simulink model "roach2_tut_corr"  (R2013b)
settings: Solver=VariableStepDiscrete  SolverMode=SingleTasking  StartTime=0.0  StopTime=100  RelTol=1e-3
undefined symbols (not defined in the file): add_latency, addr_width, Bit, bitfield, BitWidth, bram_latency, burst_size, casper_library_scopes, conv_latency, data_width, DelayLen, fan_latency, FFTSize, FFTStage, getfield, increment, led, Location, Lower, mult_latency, mux_latency, n_bits, n_bits_data, n_inputs, n_streams, n_taps, neg_latency, negate_latency, nsamples, pfb_size, pulse_len, reset_period, ROACH, ROACH2, snapshot, sx475t, sync_period, sync_period_bits, Upper, UseCounter, Width
libraries: xbsIndex_r4 x24444, casper_library_misc x73, xbsReplacements_r4 x34, casper_library_delays x14, xps_library x7
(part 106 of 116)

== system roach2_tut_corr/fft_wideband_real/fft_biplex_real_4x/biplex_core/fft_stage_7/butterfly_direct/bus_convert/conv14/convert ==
  note: (ones_bit & 1) -> round-to-even (ones_bit ^ 1) -> round-to-odd (sign_bit & 1)-> round-to-zero (sign_bit ^ 1) -> round-to-inf (X ~| 1) -> round half down (X | 1) -> round half up
  in : Inport
  Concat : xbsIndex_r4/Concat  num_inputs=2  dbl_ovrd=off  block_type=concat
  Constant : xbsIndex_r4/Constant  const=1  gui_display_data_type=Fixed-point  arith_type=Unsigned  n_bits=1  bin_pt=0  preci_type=Single  exp_width=8  frac_width=24  explicit_period=off  period=1  equ=P=C  opselect=C  inp2=PCIN>>17  opr=+  inp1=P  carry=CIN  dbl_ovrd=off  block_type=constant
  Reinterpret : xbsIndex_r4/Reinterpret  force_arith_type=on  arith_type=Unsigned  force_bin_pt=on  bin_pt=0  block_type=reinterpret
  adder : xbsIndex_r4/AddSub  mode=Addition  use_carryin=off  use_carryout=off  en=off  latency=1  precision=User Defined  arith_type="Signed  (2's comp)"  n_bits=18  bin_pt=17  quantization=Truncate  overflow=Wrap  dbl_ovrd=off  use_behavioral_HDL=off  hw_selection=Fabric  pipelined=on  use_rpm=on  block_type=addsub
  almost_half : xbsIndex_r4/Constant  const=1  gui_display_data_type=Fixed-point  arith_type=Unsigned  n_bits=19  bin_pt=0  preci_type=Single  exp_width=8  frac_width=24  explicit_period=off  period=1  equ=P=C  opselect=C  inp2=PCIN>>17  opr=+  inp1=P  carry=CIN  dbl_ovrd=off  block_type=constant
  bit : xbsIndex_r4/Slice  nbits=1  boolean_output=off  mode=Lower Bit Location + Width  bit1=0  base1=MSB of Input  bit0=1  base0=LSB of Input  dbl_ovrd=off  block_type=slice
  force1 : xbsIndex_r4/Reinterpret  force_arith_type=on  arith_type="Signed  (2's comp)"  force_bin_pt=on  bin_pt=19  block_type=reinterpret
  force2 : xbsIndex_r4/Reinterpret  force_arith_type=off  arith_type="Signed  (2's comp)"  force_bin_pt=on  bin_pt=19  block_type=reinterpret
  tweak_op : xbsIndex_r4/Logical  logical_function=AND  inputs=2  en=off  latency=0  precision=Full  arith_type=Unsigned  n_bits=8  bin_pt=2  align_bp=on  dbl_ovrd=off  block_type=logical
  out : Outport
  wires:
  tweak_op/1 -> Concat/2
  Constant/1 -> tweak_op/2
  bit/1 -> tweak_op/1
  almost_half/1 -> force2/1
  in/1 -> Reinterpret/1, bit/1
  Concat/1 -> force1/1
  Reinterpret/1 -> Concat/1
  force1/1 -> adder/1
  force2/1 -> adder/2
  adder/1 -> out/1

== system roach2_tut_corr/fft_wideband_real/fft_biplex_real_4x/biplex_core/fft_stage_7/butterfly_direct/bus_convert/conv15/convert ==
  note: (ones_bit & 1) -> round-to-even (ones_bit ^ 1) -> round-to-odd (sign_bit & 1)-> round-to-zero (sign_bit ^ 1) -> round-to-inf (X ~| 1) -> round half down (X | 1) -> round half up
  in : Inport
  Concat : xbsIndex_r4/Concat  num_inputs=2  dbl_ovrd=off  block_type=concat
  Constant : xbsIndex_r4/Constant  const=1  gui_display_data_type=Fixed-point  arith_type=Unsigned  n_bits=1  bin_pt=0  preci_type=Single  exp_width=8  frac_width=24  explicit_period=off  period=1  equ=P=C  opselect=C  inp2=PCIN>>17  opr=+  inp1=P  carry=CIN  dbl_ovrd=off  block_type=constant
  Reinterpret : xbsIndex_r4/Reinterpret  force_arith_type=on  arith_type=Unsigned  force_bin_pt=on  bin_pt=0  block_type=reinterpret
  adder : xbsIndex_r4/AddSub  mode=Addition  use_carryin=off  use_carryout=off  en=off  latency=1  precision=User Defined  arith_type="Signed  (2's comp)"  n_bits=18  bin_pt=17  quantization=Truncate  overflow=Wrap  dbl_ovrd=off  use_behavioral_HDL=off  hw_selection=Fabric  pipelined=on  use_rpm=on  block_type=addsub
  almost_half : xbsIndex_r4/Constant  const=1  gui_display_data_type=Fixed-point  arith_type=Unsigned  n_bits=19  bin_pt=0  preci_type=Single  exp_width=8  frac_width=24  explicit_period=off  period=1  equ=P=C  opselect=C  inp2=PCIN>>17  opr=+  inp1=P  carry=CIN  dbl_ovrd=off  block_type=constant
  bit : xbsIndex_r4/Slice  nbits=1  boolean_output=off  mode=Lower Bit Location + Width  bit1=0  base1=MSB of Input  bit0=1  base0=LSB of Input  dbl_ovrd=off  block_type=slice
  force1 : xbsIndex_r4/Reinterpret  force_arith_type=on  arith_type="Signed  (2's comp)"  force_bin_pt=on  bin_pt=19  block_type=reinterpret
  force2 : xbsIndex_r4/Reinterpret  force_arith_type=off  arith_type="Signed  (2's comp)"  force_bin_pt=on  bin_pt=19  block_type=reinterpret
  tweak_op : xbsIndex_r4/Logical  logical_function=AND  inputs=2  en=off  latency=0  precision=Full  arith_type=Unsigned  n_bits=8  bin_pt=2  align_bp=on  dbl_ovrd=off  block_type=logical
  out : Outport
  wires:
  tweak_op/1 -> Concat/2
  Constant/1 -> tweak_op/2
  bit/1 -> tweak_op/1
  almost_half/1 -> force2/1
  in/1 -> Reinterpret/1, bit/1
  Concat/1 -> force1/1
  Reinterpret/1 -> Concat/1
  force1/1 -> adder/1
  force2/1 -> adder/2
  adder/1 -> out/1

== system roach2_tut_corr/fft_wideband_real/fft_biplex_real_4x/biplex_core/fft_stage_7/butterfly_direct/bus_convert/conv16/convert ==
  note: (ones_bit & 1) -> round-to-even (ones_bit ^ 1) -> round-to-odd (sign_bit & 1)-> round-to-zero (sign_bit ^ 1) -> round-to-inf (X ~| 1) -> round half down (X | 1) -> round half up
  in : Inport
  Concat : xbsIndex_r4/Concat  num_inputs=2  dbl_ovrd=off  block_type=concat
  Constant : xbsIndex_r4/Constant  const=1  gui_display_data_type=Fixed-point  arith_type=Unsigned  n_bits=1  bin_pt=0  preci_type=Single  exp_width=8  frac_width=24  explicit_period=off  period=1  equ=P=C  opselect=C  inp2=PCIN>>17  opr=+  inp1=P  carry=CIN  dbl_ovrd=off  block_type=constant
  Reinterpret : xbsIndex_r4/Reinterpret  force_arith_type=on  arith_type=Unsigned  force_bin_pt=on  bin_pt=0  block_type=reinterpret
  adder : xbsIndex_r4/AddSub  mode=Addition  use_carryin=off  use_carryout=off  en=off  latency=1  precision=User Defined  arith_type="Signed  (2's comp)"  n_bits=18  bin_pt=17  quantization=Truncate  overflow=Wrap  dbl_ovrd=off  use_behavioral_HDL=off  hw_selection=Fabric  pipelined=on  use_rpm=on  block_type=addsub
  almost_half : xbsIndex_r4/Constant  const=1  gui_display_data_type=Fixed-point  arith_type=Unsigned  n_bits=19  bin_pt=0  preci_type=Single  exp_width=8  frac_width=24  explicit_period=off  period=1  equ=P=C  opselect=C  inp2=PCIN>>17  opr=+  inp1=P  carry=CIN  dbl_ovrd=off  block_type=constant
  bit : xbsIndex_r4/Slice  nbits=1  boolean_output=off  mode=Lower Bit Location + Width  bit1=0  base1=MSB of Input  bit0=1  base0=LSB of Input  dbl_ovrd=off  block_type=slice
  force1 : xbsIndex_r4/Reinterpret  force_arith_type=on  arith_type="Signed  (2's comp)"  force_bin_pt=on  bin_pt=19  block_type=reinterpret
  force2 : xbsIndex_r4/Reinterpret  force_arith_type=off  arith_type="Signed  (2's comp)"  force_bin_pt=on  bin_pt=19  block_type=reinterpret
  tweak_op : xbsIndex_r4/Logical  logical_function=AND  inputs=2  en=off  latency=0  precision=Full  arith_type=Unsigned  n_bits=8  bin_pt=2  align_bp=on  dbl_ovrd=off  block_type=logical
  out : Outport
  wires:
  tweak_op/1 -> Concat/2
  Constant/1 -> tweak_op/2
  bit/1 -> tweak_op/1
  almost_half/1 -> force2/1
  in/1 -> Reinterpret/1, bit/1
  Concat/1 -> force1/1
  Reinterpret/1 -> Concat/1
  force1/1 -> adder/1
  force2/1 -> adder/2
  adder/1 -> out/1

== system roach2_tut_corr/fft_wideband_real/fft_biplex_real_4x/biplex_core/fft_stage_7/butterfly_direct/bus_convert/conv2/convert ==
  note: (ones_bit & 1) -> round-to-even (ones_bit ^ 1) -> round-to-odd (sign_bit & 1)-> round-to-zero (sign_bit ^ 1) -> round-to-inf (X ~| 1) -> round half down (X | 1) -> round half up
  in : Inport
  Concat : xbsIndex_r4/Concat  num_inputs=2  dbl_ovrd=off  block_type=concat
  Constant : xbsIndex_r4/Constant  const=1  gui_display_data_type=Fixed-point  arith_type=Unsigned  n_bits=1  bin_pt=0  preci_type=Single  exp_width=8  frac_width=24  explicit_period=off  period=1  equ=P=C  opselect=C  inp2=PCIN>>17  opr=+  inp1=P  carry=CIN  dbl_ovrd=off  block_type=constant
  Reinterpret : xbsIndex_r4/Reinterpret  force_arith_type=on  arith_type=Unsigned  force_bin_pt=on  bin_pt=0  block_type=reinterpret
  adder : xbsIndex_r4/AddSub  mode=Addition  use_carryin=off  use_carryout=off  en=off  latency=1  precision=User Defined  arith_type="Signed  (2's comp)"  n_bits=18  bin_pt=17  quantization=Truncate  overflow=Wrap  dbl_ovrd=off  use_behavioral_HDL=off  hw_selection=Fabric  pipelined=on  use_rpm=on  block_type=addsub
  almost_half : xbsIndex_r4/Constant  const=1  gui_display_data_type=Fixed-point  arith_type=Unsigned  n_bits=19  bin_pt=0  preci_type=Single  exp_width=8  frac_width=24  explicit_period=off  period=1  equ=P=C  opselect=C  inp2=PCIN>>17  opr=+  inp1=P  carry=CIN  dbl_ovrd=off  block_type=constant
  bit : xbsIndex_r4/Slice  nbits=1  boolean_output=off  mode=Lower Bit Location + Width  bit1=0  base1=MSB of Input  bit0=1  base0=LSB of Input  dbl_ovrd=off  block_type=slice
  force1 : xbsIndex_r4/Reinterpret  force_arith_type=on  arith_type="Signed  (2's comp)"  force_bin_pt=on  bin_pt=19  block_type=reinterpret
  force2 : xbsIndex_r4/Reinterpret  force_arith_type=off  arith_type="Signed  (2's comp)"  force_bin_pt=on  bin_pt=19  block_type=reinterpret
  tweak_op : xbsIndex_r4/Logical  logical_function=AND  inputs=2  en=off  latency=0  precision=Full  arith_type=Unsigned  n_bits=8  bin_pt=2  align_bp=on  dbl_ovrd=off  block_type=logical
  out : Outport
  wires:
  tweak_op/1 -> Concat/2
  Constant/1 -> tweak_op/2
  bit/1 -> tweak_op/1
  almost_half/1 -> force2/1
  in/1 -> Reinterpret/1, bit/1
  Concat/1 -> force1/1
  Reinterpret/1 -> Concat/1
  force1/1 -> adder/1
  force2/1 -> adder/2
  adder/1 -> out/1

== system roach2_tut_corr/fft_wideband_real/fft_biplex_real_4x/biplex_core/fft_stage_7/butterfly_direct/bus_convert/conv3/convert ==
  note: (ones_bit & 1) -> round-to-even (ones_bit ^ 1) -> round-to-odd (sign_bit & 1)-> round-to-zero (sign_bit ^ 1) -> round-to-inf (X ~| 1) -> round half down (X | 1) -> round half up
  in : Inport
  Concat : xbsIndex_r4/Concat  num_inputs=2  dbl_ovrd=off  block_type=concat
  Constant : xbsIndex_r4/Constant  const=1  gui_display_data_type=Fixed-point  arith_type=Unsigned  n_bits=1  bin_pt=0  preci_type=Single  exp_width=8  frac_width=24  explicit_period=off  period=1  equ=P=C  opselect=C  inp2=PCIN>>17  opr=+  inp1=P  carry=CIN  dbl_ovrd=off  block_type=constant
  Reinterpret : xbsIndex_r4/Reinterpret  force_arith_type=on  arith_type=Unsigned  force_bin_pt=on  bin_pt=0  block_type=reinterpret
  adder : xbsIndex_r4/AddSub  mode=Addition  use_carryin=off  use_carryout=off  en=off  latency=1  precision=User Defined  arith_type="Signed  (2's comp)"  n_bits=18  bin_pt=17  quantization=Truncate  overflow=Wrap  dbl_ovrd=off  use_behavioral_HDL=off  hw_selection=Fabric  pipelined=on  use_rpm=on  block_type=addsub
  almost_half : xbsIndex_r4/Constant  const=1  gui_display_data_type=Fixed-point  arith_type=Unsigned  n_bits=19  bin_pt=0  preci_type=Single  exp_width=8  frac_width=24  explicit_period=off  period=1  equ=P=C  opselect=C  inp2=PCIN>>17  opr=+  inp1=P  carry=CIN  dbl_ovrd=off  block_type=constant
  bit : xbsIndex_r4/Slice  nbits=1  boolean_output=off  mode=Lower Bit Location + Width  bit1=0  base1=MSB of Input  bit0=1  base0=LSB of Input  dbl_ovrd=off  block_type=slice
  force1 : xbsIndex_r4/Reinterpret  force_arith_type=on  arith_type="Signed  (2's comp)"  force_bin_pt=on  bin_pt=19  block_type=reinterpret
  force2 : xbsIndex_r4/Reinterpret  force_arith_type=off  arith_type="Signed  (2's comp)"  force_bin_pt=on  bin_pt=19  block_type=reinterpret
  tweak_op : xbsIndex_r4/Logical  logical_function=AND  inputs=2  en=off  latency=0  precision=Full  arith_type=Unsigned  n_bits=8  bin_pt=2  align_bp=on  dbl_ovrd=off  block_type=logical
  out : Outport
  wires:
  tweak_op/1 -> Concat/2
  Constant/1 -> tweak_op/2
  bit/1 -> tweak_op/1
  almost_half/1 -> force2/1
  in/1 -> Reinterpret/1, bit/1
  Concat/1 -> force1/1
  Reinterpret/1 -> Concat/1
  force1/1 -> adder/1
  force2/1 -> adder/2
  adder/1 -> out/1

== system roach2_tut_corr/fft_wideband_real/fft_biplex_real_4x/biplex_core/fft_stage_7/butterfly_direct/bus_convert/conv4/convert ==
  note: (ones_bit & 1) -> round-to-even (ones_bit ^ 1) -> round-to-odd (sign_bit & 1)-> round-to-zero (sign_bit ^ 1) -> round-to-inf (X ~| 1) -> round half down (X | 1) -> round half up
  in : Inport
  Concat : xbsIndex_r4/Concat  num_inputs=2  dbl_ovrd=off  block_type=concat
  Constant : xbsIndex_r4/Constant  const=1  gui_display_data_type=Fixed-point  arith_type=Unsigned  n_bits=1  bin_pt=0  preci_type=Single  exp_width=8  frac_width=24  explicit_period=off  period=1  equ=P=C  opselect=C  inp2=PCIN>>17  opr=+  inp1=P  carry=CIN  dbl_ovrd=off  block_type=constant
  Reinterpret : xbsIndex_r4/Reinterpret  force_arith_type=on  arith_type=Unsigned  force_bin_pt=on  bin_pt=0  block_type=reinterpret
  adder : xbsIndex_r4/AddSub  mode=Addition  use_carryin=off  use_carryout=off  en=off  latency=1  precision=User Defined  arith_type="Signed  (2's comp)"  n_bits=18  bin_pt=17  quantization=Truncate  overflow=Wrap  dbl_ovrd=off  use_behavioral_HDL=off  hw_selection=Fabric  pipelined=on  use_rpm=on  block_type=addsub
  almost_half : xbsIndex_r4/Constant  const=1  gui_display_data_type=Fixed-point  arith_type=Unsigned  n_bits=19  bin_pt=0  preci_type=Single  exp_width=8  frac_width=24  explicit_period=off  period=1  equ=P=C  opselect=C  inp2=PCIN>>17  opr=+  inp1=P  carry=CIN  dbl_ovrd=off  block_type=constant
  bit : xbsIndex_r4/Slice  nbits=1  boolean_output=off  mode=Lower Bit Location + Width  bit1=0  base1=MSB of Input  bit0=1  base0=LSB of Input  dbl_ovrd=off  block_type=slice
  force1 : xbsIndex_r4/Reinterpret  force_arith_type=on  arith_type="Signed  (2's comp)"  force_bin_pt=on  bin_pt=19  block_type=reinterpret
  force2 : xbsIndex_r4/Reinterpret  force_arith_type=off  arith_type="Signed  (2's comp)"  force_bin_pt=on  bin_pt=19  block_type=reinterpret
  tweak_op : xbsIndex_r4/Logical  logical_function=AND  inputs=2  en=off  latency=0  precision=Full  arith_type=Unsigned  n_bits=8  bin_pt=2  align_bp=on  dbl_ovrd=off  block_type=logical
  out : Outport
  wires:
  tweak_op/1 -> Concat/2
  Constant/1 -> tweak_op/2
  bit/1 -> tweak_op/1
  almost_half/1 -> force2/1
  in/1 -> Reinterpret/1, bit/1
  Concat/1 -> force1/1
  Reinterpret/1 -> Concat/1
  force1/1 -> adder/1
  force2/1 -> adder/2
  adder/1 -> out/1

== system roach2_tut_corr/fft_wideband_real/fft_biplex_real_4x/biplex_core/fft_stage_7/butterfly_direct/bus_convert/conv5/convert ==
  note: (ones_bit & 1) -> round-to-even (ones_bit ^ 1) -> round-to-odd (sign_bit & 1)-> round-to-zero (sign_bit ^ 1) -> round-to-inf (X ~| 1) -> round half down (X | 1) -> round half up
  in : Inport
  Concat : xbsIndex_r4/Concat  num_inputs=2  dbl_ovrd=off  block_type=concat
  Constant : xbsIndex_r4/Constant  const=1  gui_display_data_type=Fixed-point  arith_type=Unsigned  n_bits=1  bin_pt=0  preci_type=Single  exp_width=8  frac_width=24  explicit_period=off  period=1  equ=P=C  opselect=C  inp2=PCIN>>17  opr=+  inp1=P  carry=CIN  dbl_ovrd=off  block_type=constant
  Reinterpret : xbsIndex_r4/Reinterpret  force_arith_type=on  arith_type=Unsigned  force_bin_pt=on  bin_pt=0  block_type=reinterpret
  adder : xbsIndex_r4/AddSub  mode=Addition  use_carryin=off  use_carryout=off  en=off  latency=1  precision=User Defined  arith_type="Signed  (2's comp)"  n_bits=18  bin_pt=17  quantization=Truncate  overflow=Wrap  dbl_ovrd=off  use_behavioral_HDL=off  hw_selection=Fabric  pipelined=on  use_rpm=on  block_type=addsub
  almost_half : xbsIndex_r4/Constant  const=1  gui_display_data_type=Fixed-point  arith_type=Unsigned  n_bits=19  bin_pt=0  preci_type=Single  exp_width=8  frac_width=24  explicit_period=off  period=1  equ=P=C  opselect=C  inp2=PCIN>>17  opr=+  inp1=P  carry=CIN  dbl_ovrd=off  block_type=constant
  bit : xbsIndex_r4/Slice  nbits=1  boolean_output=off  mode=Lower Bit Location + Width  bit1=0  base1=MSB of Input  bit0=1  base0=LSB of Input  dbl_ovrd=off  block_type=slice
  force1 : xbsIndex_r4/Reinterpret  force_arith_type=on  arith_type="Signed  (2's comp)"  force_bin_pt=on  bin_pt=19  block_type=reinterpret
  force2 : xbsIndex_r4/Reinterpret  force_arith_type=off  arith_type="Signed  (2's comp)"  force_bin_pt=on  bin_pt=19  block_type=reinterpret
  tweak_op : xbsIndex_r4/Logical  logical_function=AND  inputs=2  en=off  latency=0  precision=Full  arith_type=Unsigned  n_bits=8  bin_pt=2  align_bp=on  dbl_ovrd=off  block_type=logical
  out : Outport
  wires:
  tweak_op/1 -> Concat/2
  Constant/1 -> tweak_op/2
  bit/1 -> tweak_op/1
  almost_half/1 -> force2/1
  in/1 -> Reinterpret/1, bit/1
  Concat/1 -> force1/1
  Reinterpret/1 -> Concat/1
  force1/1 -> adder/1
  force2/1 -> adder/2
  adder/1 -> out/1

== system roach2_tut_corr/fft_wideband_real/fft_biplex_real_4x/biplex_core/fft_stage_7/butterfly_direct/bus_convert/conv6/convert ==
  note: (ones_bit & 1) -> round-to-even (ones_bit ^ 1) -> round-to-odd (sign_bit & 1)-> round-to-zero (sign_bit ^ 1) -> round-to-inf (X ~| 1) -> round half down (X | 1) -> round half up
  in : Inport
  Concat : xbsIndex_r4/Concat  num_inputs=2  dbl_ovrd=off  block_type=concat
  Constant : xbsIndex_r4/Constant  const=1  gui_display_data_type=Fixed-point  arith_type=Unsigned  n_bits=1  bin_pt=0  preci_type=Single  exp_width=8  frac_width=24  explicit_period=off  period=1  equ=P=C  opselect=C  inp2=PCIN>>17  opr=+  inp1=P  carry=CIN  dbl_ovrd=off  block_type=constant
  Reinterpret : xbsIndex_r4/Reinterpret  force_arith_type=on  arith_type=Unsigned  force_bin_pt=on  bin_pt=0  block_type=reinterpret
  adder : xbsIndex_r4/AddSub  mode=Addition  use_carryin=off  use_carryout=off  en=off  latency=1  precision=User Defined  arith_type="Signed  (2's comp)"  n_bits=18  bin_pt=17  quantization=Truncate  overflow=Wrap  dbl_ovrd=off  use_behavioral_HDL=off  hw_selection=Fabric  pipelined=on  use_rpm=on  block_type=addsub
  almost_half : xbsIndex_r4/Constant  const=1  gui_display_data_type=Fixed-point  arith_type=Unsigned  n_bits=19  bin_pt=0  preci_type=Single  exp_width=8  frac_width=24  explicit_period=off  period=1  equ=P=C  opselect=C  inp2=PCIN>>17  opr=+  inp1=P  carry=CIN  dbl_ovrd=off  block_type=constant
  bit : xbsIndex_r4/Slice  nbits=1  boolean_output=off  mode=Lower Bit Location + Width  bit1=0  base1=MSB of Input  bit0=1  base0=LSB of Input  dbl_ovrd=off  block_type=slice
  force1 : xbsIndex_r4/Reinterpret  force_arith_type=on  arith_type="Signed  (2's comp)"  force_bin_pt=on  bin_pt=19  block_type=reinterpret
  force2 : xbsIndex_r4/Reinterpret  force_arith_type=off  arith_type="Signed  (2's comp)"  force_bin_pt=on  bin_pt=19  block_type=reinterpret
  tweak_op : xbsIndex_r4/Logical  logical_function=AND  inputs=2  en=off  latency=0  precision=Full  arith_type=Unsigned  n_bits=8  bin_pt=2  align_bp=on  dbl_ovrd=off  block_type=logical
  out : Outport
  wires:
  tweak_op/1 -> Concat/2
  Constant/1 -> tweak_op/2
  bit/1 -> tweak_op/1
  almost_half/1 -> force2/1
  in/1 -> Reinterpret/1, bit/1
  Concat/1 -> force1/1
  Reinterpret/1 -> Concat/1
  force1/1 -> adder/1
  force2/1 -> adder/2
  adder/1 -> out/1

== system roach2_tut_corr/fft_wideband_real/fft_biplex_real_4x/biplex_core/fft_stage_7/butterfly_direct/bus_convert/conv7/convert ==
  note: (ones_bit & 1) -> round-to-even (ones_bit ^ 1) -> round-to-odd (sign_bit & 1)-> round-to-zero (sign_bit ^ 1) -> round-to-inf (X ~| 1) -> round half down (X | 1) -> round half up
  in : Inport
  Concat : xbsIndex_r4/Concat  num_inputs=2  dbl_ovrd=off  block_type=concat
  Constant : xbsIndex_r4/Constant  const=1  gui_display_data_type=Fixed-point  arith_type=Unsigned  n_bits=1  bin_pt=0  preci_type=Single  exp_width=8  frac_width=24  explicit_period=off  period=1  equ=P=C  opselect=C  inp2=PCIN>>17  opr=+  inp1=P  carry=CIN  dbl_ovrd=off  block_type=constant
  Reinterpret : xbsIndex_r4/Reinterpret  force_arith_type=on  arith_type=Unsigned  force_bin_pt=on  bin_pt=0  block_type=reinterpret
  adder : xbsIndex_r4/AddSub  mode=Addition  use_carryin=off  use_carryout=off  en=off  latency=1  precision=User Defined  arith_type="Signed  (2's comp)"  n_bits=18  bin_pt=17  quantization=Truncate  overflow=Wrap  dbl_ovrd=off  use_behavioral_HDL=off  hw_selection=Fabric  pipelined=on  use_rpm=on  block_type=addsub
  almost_half : xbsIndex_r4/Constant  const=1  gui_display_data_type=Fixed-point  arith_type=Unsigned  n_bits=19  bin_pt=0  preci_type=Single  exp_width=8  frac_width=24  explicit_period=off  period=1  equ=P=C  opselect=C  inp2=PCIN>>17  opr=+  inp1=P  carry=CIN  dbl_ovrd=off  block_type=constant
  bit : xbsIndex_r4/Slice  nbits=1  boolean_output=off  mode=Lower Bit Location + Width  bit1=0  base1=MSB of Input  bit0=1  base0=LSB of Input  dbl_ovrd=off  block_type=slice
  force1 : xbsIndex_r4/Reinterpret  force_arith_type=on  arith_type="Signed  (2's comp)"  force_bin_pt=on  bin_pt=19  block_type=reinterpret
  force2 : xbsIndex_r4/Reinterpret  force_arith_type=off  arith_type="Signed  (2's comp)"  force_bin_pt=on  bin_pt=19  block_type=reinterpret
  tweak_op : xbsIndex_r4/Logical  logical_function=AND  inputs=2  en=off  latency=0  precision=Full  arith_type=Unsigned  n_bits=8  bin_pt=2  align_bp=on  dbl_ovrd=off  block_type=logical
  out : Outport
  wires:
  tweak_op/1 -> Concat/2
  Constant/1 -> tweak_op/2
  bit/1 -> tweak_op/1
  almost_half/1 -> force2/1
  in/1 -> Reinterpret/1, bit/1
  Concat/1 -> force1/1
  Reinterpret/1 -> Concat/1
  force1/1 -> adder/1
  force2/1 -> adder/2
  adder/1 -> out/1

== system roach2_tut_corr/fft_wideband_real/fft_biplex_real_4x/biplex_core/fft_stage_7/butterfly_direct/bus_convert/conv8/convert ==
  note: (ones_bit & 1) -> round-to-even (ones_bit ^ 1) -> round-to-odd (sign_bit & 1)-> round-to-zero (sign_bit ^ 1) -> round-to-inf (X ~| 1) -> round half down (X | 1) -> round half up
  in : Inport
  Concat : xbsIndex_r4/Concat  num_inputs=2  dbl_ovrd=off  block_type=concat
  Constant : xbsIndex_r4/Constant  const=1  gui_display_data_type=Fixed-point  arith_type=Unsigned  n_bits=1  bin_pt=0  preci_type=Single  exp_width=8  frac_width=24  explicit_period=off  period=1  equ=P=C  opselect=C  inp2=PCIN>>17  opr=+  inp1=P  carry=CIN  dbl_ovrd=off  block_type=constant
  Reinterpret : xbsIndex_r4/Reinterpret  force_arith_type=on  arith_type=Unsigned  force_bin_pt=on  bin_pt=0  block_type=reinterpret
  adder : xbsIndex_r4/AddSub  mode=Addition  use_carryin=off  use_carryout=off  en=off  latency=1  precision=User Defined  arith_type="Signed  (2's comp)"  n_bits=18  bin_pt=17  quantization=Truncate  overflow=Wrap  dbl_ovrd=off  use_behavioral_HDL=off  hw_selection=Fabric  pipelined=on  use_rpm=on  block_type=addsub
  almost_half : xbsIndex_r4/Constant  const=1  gui_display_data_type=Fixed-point  arith_type=Unsigned  n_bits=19  bin_pt=0  preci_type=Single  exp_width=8  frac_width=24  explicit_period=off  period=1  equ=P=C  opselect=C  inp2=PCIN>>17  opr=+  inp1=P  carry=CIN  dbl_ovrd=off  block_type=constant
  bit : xbsIndex_r4/Slice  nbits=1  boolean_output=off  mode=Lower Bit Location + Width  bit1=0  base1=MSB of Input  bit0=1  base0=LSB of Input  dbl_ovrd=off  block_type=slice
  force1 : xbsIndex_r4/Reinterpret  force_arith_type=on  arith_type="Signed  (2's comp)"  force_bin_pt=on  bin_pt=19  block_type=reinterpret
  force2 : xbsIndex_r4/Reinterpret  force_arith_type=off  arith_type="Signed  (2's comp)"  force_bin_pt=on  bin_pt=19  block_type=reinterpret
  tweak_op : xbsIndex_r4/Logical  logical_function=AND  inputs=2  en=off  latency=0  precision=Full  arith_type=Unsigned  n_bits=8  bin_pt=2  align_bp=on  dbl_ovrd=off  block_type=logical
  out : Outport
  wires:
  tweak_op/1 -> Concat/2
  Constant/1 -> tweak_op/2
  bit/1 -> tweak_op/1
  almost_half/1 -> force2/1
  in/1 -> Reinterpret/1, bit/1
  Concat/1 -> force1/1
  Reinterpret/1 -> Concat/1
  force1/1 -> adder/1
  force2/1 -> adder/2
  adder/1 -> out/1

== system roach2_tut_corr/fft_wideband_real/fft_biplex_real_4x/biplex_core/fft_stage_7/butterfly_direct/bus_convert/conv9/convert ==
  note: (ones_bit & 1) -> round-to-even (ones_bit ^ 1) -> round-to-odd (sign_bit & 1)-> round-to-zero (sign_bit ^ 1) -> round-to-inf (X ~| 1) -> round half down (X | 1) -> round half up
  in : Inport
  Concat : xbsIndex_r4/Concat  num_inputs=2  dbl_ovrd=off  block_type=concat
  Constant : xbsIndex_r4/Constant  const=1  gui_display_data_type=Fixed-point  arith_type=Unsigned  n_bits=1  bin_pt=0  preci_type=Single  exp_width=8  frac_width=24  explicit_period=off  period=1  equ=P=C  opselect=C  inp2=PCIN>>17  opr=+  inp1=P  carry=CIN  dbl_ovrd=off  block_type=constant
  Reinterpret : xbsIndex_r4/Reinterpret  force_arith_type=on  arith_type=Unsigned  force_bin_pt=on  bin_pt=0  block_type=reinterpret
  adder : xbsIndex_r4/AddSub  mode=Addition  use_carryin=off  use_carryout=off  en=off  latency=1  precision=User Defined  arith_type="Signed  (2's comp)"  n_bits=18  bin_pt=17  quantization=Truncate  overflow=Wrap  dbl_ovrd=off  use_behavioral_HDL=off  hw_selection=Fabric  pipelined=on  use_rpm=on  block_type=addsub
  almost_half : xbsIndex_r4/Constant  const=1  gui_display_data_type=Fixed-point  arith_type=Unsigned  n_bits=19  bin_pt=0  preci_type=Single  exp_width=8  frac_width=24  explicit_period=off  period=1  equ=P=C  opselect=C  inp2=PCIN>>17  opr=+  inp1=P  carry=CIN  dbl_ovrd=off  block_type=constant
  bit : xbsIndex_r4/Slice  nbits=1  boolean_output=off  mode=Lower Bit Location + Width  bit1=0  base1=MSB of Input  bit0=1  base0=LSB of Input  dbl_ovrd=off  block_type=slice
  force1 : xbsIndex_r4/Reinterpret  force_arith_type=on  arith_type="Signed  (2's comp)"  force_bin_pt=on  bin_pt=19  block_type=reinterpret
  force2 : xbsIndex_r4/Reinterpret  force_arith_type=off  arith_type="Signed  (2's comp)"  force_bin_pt=on  bin_pt=19  block_type=reinterpret
  tweak_op : xbsIndex_r4/Logical  logical_function=AND  inputs=2  en=off  latency=0  precision=Full  arith_type=Unsigned  n_bits=8  bin_pt=2  align_bp=on  dbl_ovrd=off  block_type=logical
  out : Outport
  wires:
  tweak_op/1 -> Concat/2
  Constant/1 -> tweak_op/2
  bit/1 -> tweak_op/1
  almost_half/1 -> force2/1
  in/1 -> Reinterpret/1, bit/1
  Concat/1 -> force1/1
  Reinterpret/1 -> Concat/1
  force1/1 -> adder/1
  force2/1 -> adder/2
  adder/1 -> out/1

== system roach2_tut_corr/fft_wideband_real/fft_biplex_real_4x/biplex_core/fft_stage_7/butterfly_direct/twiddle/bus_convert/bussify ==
  in1 : Inport
  in2 : Inport  Port=2
  in3 : Inport  Port=3
  in4 : Inport  Port=4
  in5 : Inport  Port=5
  in6 : Inport  Port=6
  in7 : Inport  Port=7
  in8 : Inport  Port=8
  concatenate : xbsIndex_r4/Concat  num_inputs=8  dbl_ovrd=off  block_type=concat
  reinterpret{1..8} (8 alike) : xbsIndex_r4/Reinterpret  force_arith_type=on  arith_type=Unsigned  force_bin_pt=on  bin_pt=0  block_type=reinterpret
  bus_out : Outport
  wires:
  concatenate/1 -> bus_out/1
  in1/1 -> reinterpret1/1
  reinterpret1/1 -> concatenate/1
  in2/1 -> reinterpret2/1
  reinterpret2/1 -> concatenate/2
  in3/1 -> reinterpret3/1
  reinterpret3/1 -> concatenate/3
  in4/1 -> reinterpret4/1
  reinterpret4/1 -> concatenate/4
  in5/1 -> reinterpret5/1
  reinterpret5/1 -> concatenate/5
  in6/1 -> reinterpret6/1
  reinterpret6/1 -> concatenate/6
  in7/1 -> reinterpret7/1
  reinterpret7/1 -> concatenate/7
  in8/1 -> reinterpret8/1
  reinterpret8/1 -> concatenate/8

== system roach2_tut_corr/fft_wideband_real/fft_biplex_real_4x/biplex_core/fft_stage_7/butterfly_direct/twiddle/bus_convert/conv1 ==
  note: (ones_bit & 1) -> round-to-even (ones_bit ^ 1) -> round-to-odd (sign_bit & 1)-> round-to-zero (sign_bit ^ 1) -> round-to-inf (X ~| 1) -> round half down (X | 1) -> round half up
  in : Inport
  Concat : xbsIndex_r4/Concat  num_inputs=2  dbl_ovrd=off  block_type=concat
  Constant : xbsIndex_r4/Constant  const=1  gui_display_data_type=Fixed-point  arith_type=Unsigned  n_bits=1  bin_pt=0  preci_type=Single  exp_width=8  frac_width=24  explicit_period=off  period=1  equ=P=C  opselect=C  inp2=PCIN>>17  opr=+  inp1=P  carry=CIN  dbl_ovrd=off  block_type=constant
  Reinterpret : xbsIndex_r4/Reinterpret  force_arith_type=on  arith_type=Unsigned  force_bin_pt=on  bin_pt=0  block_type=reinterpret
  adder : xbsIndex_r4/AddSub  mode=Addition  use_carryin=off  use_carryout=off  en=off  latency=1  precision=User Defined  arith_type="Signed  (2's comp)"  n_bits=19  bin_pt=17  quantization=Truncate  overflow=Wrap  dbl_ovrd=off  use_behavioral_HDL=off  hw_selection=Fabric  pipelined=on  use_rpm=on  block_type=addsub
  almost_half : xbsIndex_r4/Constant  const=131071  gui_display_data_type=Fixed-point  arith_type=Unsigned  n_bits=35  bin_pt=0  preci_type=Single  exp_width=8  frac_width=24  explicit_period=off  period=1  equ=P=C  opselect=C  inp2=PCIN>>17  opr=+  inp1=P  carry=CIN  dbl_ovrd=off  block_type=constant
  bit : xbsIndex_r4/Slice  nbits=1  boolean_output=off  mode=Lower Bit Location + Width  bit1=0  base1=MSB of Input  bit0=17  base0=LSB of Input  dbl_ovrd=off  block_type=slice
  force1 : xbsIndex_r4/Reinterpret  force_arith_type=on  arith_type="Signed  (2's comp)"  force_bin_pt=on  bin_pt=35  block_type=reinterpret
  force2 : xbsIndex_r4/Reinterpret  force_arith_type=off  arith_type="Signed  (2's comp)"  force_bin_pt=on  bin_pt=35  block_type=reinterpret
  tweak_op : xbsIndex_r4/Logical  logical_function=AND  inputs=2  en=off  latency=0  precision=Full  arith_type=Unsigned  n_bits=8  bin_pt=2  align_bp=on  dbl_ovrd=off  block_type=logical
  out : Outport
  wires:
  tweak_op/1 -> Concat/2
  Constant/1 -> tweak_op/2
  bit/1 -> tweak_op/1
  almost_half/1 -> force2/1
  in/1 -> Reinterpret/1, bit/1
  Concat/1 -> force1/1
  Reinterpret/1 -> Concat/1
  force1/1 -> adder/1
  force2/1 -> adder/2
  adder/1 -> out/1

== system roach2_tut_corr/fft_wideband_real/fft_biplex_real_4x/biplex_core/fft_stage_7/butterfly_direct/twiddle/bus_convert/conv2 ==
  note: (ones_bit & 1) -> round-to-even (ones_bit ^ 1) -> round-to-odd (sign_bit & 1)-> round-to-zero (sign_bit ^ 1) -> round-to-inf (X ~| 1) -> round half down (X | 1) -> round half up
  in : Inport
  Concat : xbsIndex_r4/Concat  num_inputs=2  dbl_ovrd=off  block_type=concat
  Constant : xbsIndex_r4/Constant  const=1  gui_display_data_type=Fixed-point  arith_type=Unsigned  n_bits=1  bin_pt=0  preci_type=Single  exp_width=8  frac_width=24  explicit_period=off  period=1  equ=P=C  opselect=C  inp2=PCIN>>17  opr=+  inp1=P  carry=CIN  dbl_ovrd=off  block_type=constant
  Reinterpret : xbsIndex_r4/Reinterpret  force_arith_type=on  arith_type=Unsigned  force_bin_pt=on  bin_pt=0  block_type=reinterpret
  adder : xbsIndex_r4/AddSub  mode=Addition  use_carryin=off  use_carryout=off  en=off  latency=1  precision=User Defined  arith_type="Signed  (2's comp)"  n_bits=19  bin_pt=17  quantization=Truncate  overflow=Wrap  dbl_ovrd=off  use_behavioral_HDL=off  hw_selection=Fabric  pipelined=on  use_rpm=on  block_type=addsub
  almost_half : xbsIndex_r4/Constant  const=131071  gui_display_data_type=Fixed-point  arith_type=Unsigned  n_bits=35  bin_pt=0  preci_type=Single  exp_width=8  frac_width=24  explicit_period=off  period=1  equ=P=C  opselect=C  inp2=PCIN>>17  opr=+  inp1=P  carry=CIN  dbl_ovrd=off  block_type=constant
  bit : xbsIndex_r4/Slice  nbits=1  boolean_output=off  mode=Lower Bit Location + Width  bit1=0  base1=MSB of Input  bit0=17  base0=LSB of Input  dbl_ovrd=off  block_type=slice
  force1 : xbsIndex_r4/Reinterpret  force_arith_type=on  arith_type="Signed  (2's comp)"  force_bin_pt=on  bin_pt=35  block_type=reinterpret
  force2 : xbsIndex_r4/Reinterpret  force_arith_type=off  arith_type="Signed  (2's comp)"  force_bin_pt=on  bin_pt=35  block_type=reinterpret
  tweak_op : xbsIndex_r4/Logical  logical_function=AND  inputs=2  en=off  latency=0  precision=Full  arith_type=Unsigned  n_bits=8  bin_pt=2  align_bp=on  dbl_ovrd=off  block_type=logical
  out : Outport
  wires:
  tweak_op/1 -> Concat/2
  Constant/1 -> tweak_op/2
  bit/1 -> tweak_op/1
  almost_half/1 -> force2/1
  in/1 -> Reinterpret/1, bit/1
  Concat/1 -> force1/1
  Reinterpret/1 -> Concat/1
  force1/1 -> adder/1
  force2/1 -> adder/2
  adder/1 -> out/1

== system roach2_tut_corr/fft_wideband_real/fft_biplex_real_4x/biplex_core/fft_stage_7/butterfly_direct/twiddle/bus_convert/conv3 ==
  note: (ones_bit & 1) -> round-to-even (ones_bit ^ 1) -> round-to-odd (sign_bit & 1)-> round-to-zero (sign_bit ^ 1) -> round-to-inf (X ~| 1) -> round half down (X | 1) -> round half up
  in : Inport
  Concat : xbsIndex_r4/Concat  num_inputs=2  dbl_ovrd=off  block_type=concat
  Constant : xbsIndex_r4/Constant  const=1  gui_display_data_type=Fixed-point  arith_type=Unsigned  n_bits=1  bin_pt=0  preci_type=Single  exp_width=8  frac_width=24  explicit_period=off  period=1  equ=P=C  opselect=C  inp2=PCIN>>17  opr=+  inp1=P  carry=CIN  dbl_ovrd=off  block_type=constant
  Reinterpret : xbsIndex_r4/Reinterpret  force_arith_type=on  arith_type=Unsigned  force_bin_pt=on  bin_pt=0  block_type=reinterpret
  adder : xbsIndex_r4/AddSub  mode=Addition  use_carryin=off  use_carryout=off  en=off  latency=1  precision=User Defined  arith_type="Signed  (2's comp)"  n_bits=19  bin_pt=17  quantization=Truncate  overflow=Wrap  dbl_ovrd=off  use_behavioral_HDL=off  hw_selection=Fabric  pipelined=on  use_rpm=on  block_type=addsub
  almost_half : xbsIndex_r4/Constant  const=131071  gui_display_data_type=Fixed-point  arith_type=Unsigned  n_bits=35  bin_pt=0  preci_type=Single  exp_width=8  frac_width=24  explicit_period=off  period=1  equ=P=C  opselect=C  inp2=PCIN>>17  opr=+  inp1=P  carry=CIN  dbl_ovrd=off  block_type=constant
  bit : xbsIndex_r4/Slice  nbits=1  boolean_output=off  mode=Lower Bit Location + Width  bit1=0  base1=MSB of Input  bit0=17  base0=LSB of Input  dbl_ovrd=off  block_type=slice
  force1 : xbsIndex_r4/Reinterpret  force_arith_type=on  arith_type="Signed  (2's comp)"  force_bin_pt=on  bin_pt=35  block_type=reinterpret
  force2 : xbsIndex_r4/Reinterpret  force_arith_type=off  arith_type="Signed  (2's comp)"  force_bin_pt=on  bin_pt=35  block_type=reinterpret
  tweak_op : xbsIndex_r4/Logical  logical_function=AND  inputs=2  en=off  latency=0  precision=Full  arith_type=Unsigned  n_bits=8  bin_pt=2  align_bp=on  dbl_ovrd=off  block_type=logical
  out : Outport
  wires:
  tweak_op/1 -> Concat/2
  Constant/1 -> tweak_op/2
  bit/1 -> tweak_op/1
  almost_half/1 -> force2/1
  in/1 -> Reinterpret/1, bit/1
  Concat/1 -> force1/1
  Reinterpret/1 -> Concat/1
  force1/1 -> adder/1
  force2/1 -> adder/2
  adder/1 -> out/1

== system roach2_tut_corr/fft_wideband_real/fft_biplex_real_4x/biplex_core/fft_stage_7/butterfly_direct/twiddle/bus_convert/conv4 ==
  note: (ones_bit & 1) -> round-to-even (ones_bit ^ 1) -> round-to-odd (sign_bit & 1)-> round-to-zero (sign_bit ^ 1) -> round-to-inf (X ~| 1) -> round half down (X | 1) -> round half up
  in : Inport
  Concat : xbsIndex_r4/Concat  num_inputs=2  dbl_ovrd=off  block_type=concat
  Constant : xbsIndex_r4/Constant  const=1  gui_display_data_type=Fixed-point  arith_type=Unsigned  n_bits=1  bin_pt=0  preci_type=Single  exp_width=8  frac_width=24  explicit_period=off  period=1  equ=P=C  opselect=C  inp2=PCIN>>17  opr=+  inp1=P  carry=CIN  dbl_ovrd=off  block_type=constant
  Reinterpret : xbsIndex_r4/Reinterpret  force_arith_type=on  arith_type=Unsigned  force_bin_pt=on  bin_pt=0  block_type=reinterpret
  adder : xbsIndex_r4/AddSub  mode=Addition  use_carryin=off  use_carryout=off  en=off  latency=1  precision=User Defined  arith_type="Signed  (2's comp)"  n_bits=19  bin_pt=17  quantization=Truncate  overflow=Wrap  dbl_ovrd=off  use_behavioral_HDL=off  hw_selection=Fabric  pipelined=on  use_rpm=on  block_type=addsub
  almost_half : xbsIndex_r4/Constant  const=131071  gui_display_data_type=Fixed-point  arith_type=Unsigned  n_bits=35  bin_pt=0  preci_type=Single  exp_width=8  frac_width=24  explicit_period=off  period=1  equ=P=C  opselect=C  inp2=PCIN>>17  opr=+  inp1=P  carry=CIN  dbl_ovrd=off  block_type=constant
  bit : xbsIndex_r4/Slice  nbits=1  boolean_output=off  mode=Lower Bit Location + Width  bit1=0  base1=MSB of Input  bit0=17  base0=LSB of Input  dbl_ovrd=off  block_type=slice
  force1 : xbsIndex_r4/Reinterpret  force_arith_type=on  arith_type="Signed  (2's comp)"  force_bin_pt=on  bin_pt=35  block_type=reinterpret
  force2 : xbsIndex_r4/Reinterpret  force_arith_type=off  arith_type="Signed  (2's comp)"  force_bin_pt=on  bin_pt=35  block_type=reinterpret
  tweak_op : xbsIndex_r4/Logical  logical_function=AND  inputs=2  en=off  latency=0  precision=Full  arith_type=Unsigned  n_bits=8  bin_pt=2  align_bp=on  dbl_ovrd=off  block_type=logical
  out : Outport
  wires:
  tweak_op/1 -> Concat/2
  Constant/1 -> tweak_op/2
  bit/1 -> tweak_op/1
  almost_half/1 -> force2/1
  in/1 -> Reinterpret/1, bit/1
  Concat/1 -> force1/1
  Reinterpret/1 -> Concat/1
  force1/1 -> adder/1
  force2/1 -> adder/2
  adder/1 -> out/1

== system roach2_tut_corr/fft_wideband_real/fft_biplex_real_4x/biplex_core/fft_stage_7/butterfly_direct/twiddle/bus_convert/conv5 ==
  note: (ones_bit & 1) -> round-to-even (ones_bit ^ 1) -> round-to-odd (sign_bit & 1)-> round-to-zero (sign_bit ^ 1) -> round-to-inf (X ~| 1) -> round half down (X | 1) -> round half up
  in : Inport
  Concat : xbsIndex_r4/Concat  num_inputs=2  dbl_ovrd=off  block_type=concat
  Constant : xbsIndex_r4/Constant  const=1  gui_display_data_type=Fixed-point  arith_type=Unsigned  n_bits=1  bin_pt=0  preci_type=Single  exp_width=8  frac_width=24  explicit_period=off  period=1  equ=P=C  opselect=C  inp2=PCIN>>17  opr=+  inp1=P  carry=CIN  dbl_ovrd=off  block_type=constant
  Reinterpret : xbsIndex_r4/Reinterpret  force_arith_type=on  arith_type=Unsigned  force_bin_pt=on  bin_pt=0  block_type=reinterpret
  adder : xbsIndex_r4/AddSub  mode=Addition  use_carryin=off  use_carryout=off  en=off  latency=1  precision=User Defined  arith_type="Signed  (2's comp)"  n_bits=19  bin_pt=17  quantization=Truncate  overflow=Wrap  dbl_ovrd=off  use_behavioral_HDL=off  hw_selection=Fabric  pipelined=on  use_rpm=on  block_type=addsub
  almost_half : xbsIndex_r4/Constant  const=131071  gui_display_data_type=Fixed-point  arith_type=Unsigned  n_bits=35  bin_pt=0  preci_type=Single  exp_width=8  frac_width=24  explicit_period=off  period=1  equ=P=C  opselect=C  inp2=PCIN>>17  opr=+  inp1=P  carry=CIN  dbl_ovrd=off  block_type=constant
  bit : xbsIndex_r4/Slice  nbits=1  boolean_output=off  mode=Lower Bit Location + Width  bit1=0  base1=MSB of Input  bit0=17  base0=LSB of Input  dbl_ovrd=off  block_type=slice
  force1 : xbsIndex_r4/Reinterpret  force_arith_type=on  arith_type="Signed  (2's comp)"  force_bin_pt=on  bin_pt=35  block_type=reinterpret
  force2 : xbsIndex_r4/Reinterpret  force_arith_type=off  arith_type="Signed  (2's comp)"  force_bin_pt=on  bin_pt=35  block_type=reinterpret
  tweak_op : xbsIndex_r4/Logical  logical_function=AND  inputs=2  en=off  latency=0  precision=Full  arith_type=Unsigned  n_bits=8  bin_pt=2  align_bp=on  dbl_ovrd=off  block_type=logical
  out : Outport
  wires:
  tweak_op/1 -> Concat/2
  Constant/1 -> tweak_op/2
  bit/1 -> tweak_op/1
  almost_half/1 -> force2/1
  in/1 -> Reinterpret/1, bit/1
  Concat/1 -> force1/1
  Reinterpret/1 -> Concat/1
  force1/1 -> adder/1
  force2/1 -> adder/2
  adder/1 -> out/1

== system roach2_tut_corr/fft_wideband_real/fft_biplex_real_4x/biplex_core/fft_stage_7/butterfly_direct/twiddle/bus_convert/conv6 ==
  note: (ones_bit & 1) -> round-to-even (ones_bit ^ 1) -> round-to-odd (sign_bit & 1)-> round-to-zero (sign_bit ^ 1) -> round-to-inf (X ~| 1) -> round half down (X | 1) -> round half up
  in : Inport
  Concat : xbsIndex_r4/Concat  num_inputs=2  dbl_ovrd=off  block_type=concat
  Constant : xbsIndex_r4/Constant  const=1  gui_display_data_type=Fixed-point  arith_type=Unsigned  n_bits=1  bin_pt=0  preci_type=Single  exp_width=8  frac_width=24  explicit_period=off  period=1  equ=P=C  opselect=C  inp2=PCIN>>17  opr=+  inp1=P  carry=CIN  dbl_ovrd=off  block_type=constant
  Reinterpret : xbsIndex_r4/Reinterpret  force_arith_type=on  arith_type=Unsigned  force_bin_pt=on  bin_pt=0  block_type=reinterpret
  adder : xbsIndex_r4/AddSub  mode=Addition  use_carryin=off  use_carryout=off  en=off  latency=1  precision=User Defined  arith_type="Signed  (2's comp)"  n_bits=19  bin_pt=17  quantization=Truncate  overflow=Wrap  dbl_ovrd=off  use_behavioral_HDL=off  hw_selection=Fabric  pipelined=on  use_rpm=on  block_type=addsub
  almost_half : xbsIndex_r4/Constant  const=131071  gui_display_data_type=Fixed-point  arith_type=Unsigned  n_bits=35  bin_pt=0  preci_type=Single  exp_width=8  frac_width=24  explicit_period=off  period=1  equ=P=C  opselect=C  inp2=PCIN>>17  opr=+  inp1=P  carry=CIN  dbl_ovrd=off  block_type=constant
  bit : xbsIndex_r4/Slice  nbits=1  boolean_output=off  mode=Lower Bit Location + Width  bit1=0  base1=MSB of Input  bit0=17  base0=LSB of Input  dbl_ovrd=off  block_type=slice
  force1 : xbsIndex_r4/Reinterpret  force_arith_type=on  arith_type="Signed  (2's comp)"  force_bin_pt=on  bin_pt=35  block_type=reinterpret
  force2 : xbsIndex_r4/Reinterpret  force_arith_type=off  arith_type="Signed  (2's comp)"  force_bin_pt=on  bin_pt=35  block_type=reinterpret
  tweak_op : xbsIndex_r4/Logical  logical_function=AND  inputs=2  en=off  latency=0  precision=Full  arith_type=Unsigned  n_bits=8  bin_pt=2  align_bp=on  dbl_ovrd=off  block_type=logical
  out : Outport
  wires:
  tweak_op/1 -> Concat/2
  Constant/1 -> tweak_op/2
  bit/1 -> tweak_op/1
  almost_half/1 -> force2/1
  in/1 -> Reinterpret/1, bit/1
  Concat/1 -> force1/1
  Reinterpret/1 -> Concat/1
  force1/1 -> adder/1
  force2/1 -> adder/2
  adder/1 -> out/1

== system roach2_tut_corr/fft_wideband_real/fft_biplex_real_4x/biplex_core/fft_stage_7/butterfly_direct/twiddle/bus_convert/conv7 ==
  note: (ones_bit & 1) -> round-to-even (ones_bit ^ 1) -> round-to-odd (sign_bit & 1)-> round-to-zero (sign_bit ^ 1) -> round-to-inf (X ~| 1) -> round half down (X | 1) -> round half up
  in : Inport
  Concat : xbsIndex_r4/Concat  num_inputs=2  dbl_ovrd=off  block_type=concat
  Constant : xbsIndex_r4/Constant  const=1  gui_display_data_type=Fixed-point  arith_type=Unsigned  n_bits=1  bin_pt=0  preci_type=Single  exp_width=8  frac_width=24  explicit_period=off  period=1  equ=P=C  opselect=C  inp2=PCIN>>17  opr=+  inp1=P  carry=CIN  dbl_ovrd=off  block_type=constant
  Reinterpret : xbsIndex_r4/Reinterpret  force_arith_type=on  arith_type=Unsigned  force_bin_pt=on  bin_pt=0  block_type=reinterpret
  adder : xbsIndex_r4/AddSub  mode=Addition  use_carryin=off  use_carryout=off  en=off  latency=1  precision=User Defined  arith_type="Signed  (2's comp)"  n_bits=19  bin_pt=17  quantization=Truncate  overflow=Wrap  dbl_ovrd=off  use_behavioral_HDL=off  hw_selection=Fabric  pipelined=on  use_rpm=on  block_type=addsub
  almost_half : xbsIndex_r4/Constant  const=131071  gui_display_data_type=Fixed-point  arith_type=Unsigned  n_bits=35  bin_pt=0  preci_type=Single  exp_width=8  frac_width=24  explicit_period=off  period=1  equ=P=C  opselect=C  inp2=PCIN>>17  opr=+  inp1=P  carry=CIN  dbl_ovrd=off  block_type=constant
  bit : xbsIndex_r4/Slice  nbits=1  boolean_output=off  mode=Lower Bit Location + Width  bit1=0  base1=MSB of Input  bit0=17  base0=LSB of Input  dbl_ovrd=off  block_type=slice
  force1 : xbsIndex_r4/Reinterpret  force_arith_type=on  arith_type="Signed  (2's comp)"  force_bin_pt=on  bin_pt=35  block_type=reinterpret
  force2 : xbsIndex_r4/Reinterpret  force_arith_type=off  arith_type="Signed  (2's comp)"  force_bin_pt=on  bin_pt=35  block_type=reinterpret
  tweak_op : xbsIndex_r4/Logical  logical_function=AND  inputs=2  en=off  latency=0  precision=Full  arith_type=Unsigned  n_bits=8  bin_pt=2  align_bp=on  dbl_ovrd=off  block_type=logical
  out : Outport
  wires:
  tweak_op/1 -> Concat/2
  Constant/1 -> tweak_op/2
  bit/1 -> tweak_op/1
  almost_half/1 -> force2/1
  in/1 -> Reinterpret/1, bit/1
  Concat/1 -> force1/1
  Reinterpret/1 -> Concat/1
  force1/1 -> adder/1
  force2/1 -> adder/2
  adder/1 -> out/1

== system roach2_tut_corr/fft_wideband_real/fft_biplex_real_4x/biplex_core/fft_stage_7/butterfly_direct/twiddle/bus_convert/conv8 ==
  note: (ones_bit & 1) -> round-to-even (ones_bit ^ 1) -> round-to-odd (sign_bit & 1)-> round-to-zero (sign_bit ^ 1) -> round-to-inf (X ~| 1) -> round half down (X | 1) -> round half up
  in : Inport
  Concat : xbsIndex_r4/Concat  num_inputs=2  dbl_ovrd=off  block_type=concat
  Constant : xbsIndex_r4/Constant  const=1  gui_display_data_type=Fixed-point  arith_type=Unsigned  n_bits=1  bin_pt=0  preci_type=Single  exp_width=8  frac_width=24  explicit_period=off  period=1  equ=P=C  opselect=C  inp2=PCIN>>17  opr=+  inp1=P  carry=CIN  dbl_ovrd=off  block_type=constant
  Reinterpret : xbsIndex_r4/Reinterpret  force_arith_type=on  arith_type=Unsigned  force_bin_pt=on  bin_pt=0  block_type=reinterpret
  adder : xbsIndex_r4/AddSub  mode=Addition  use_carryin=off  use_carryout=off  en=off  latency=1  precision=User Defined  arith_type="Signed  (2's comp)"  n_bits=19  bin_pt=17  quantization=Truncate  overflow=Wrap  dbl_ovrd=off  use_behavioral_HDL=off  hw_selection=Fabric  pipelined=on  use_rpm=on  block_type=addsub
  almost_half : xbsIndex_r4/Constant  const=131071  gui_display_data_type=Fixed-point  arith_type=Unsigned  n_bits=35  bin_pt=0  preci_type=Single  exp_width=8  frac_width=24  explicit_period=off  period=1  equ=P=C  opselect=C  inp2=PCIN>>17  opr=+  inp1=P  carry=CIN  dbl_ovrd=off  block_type=constant
  bit : xbsIndex_r4/Slice  nbits=1  boolean_output=off  mode=Lower Bit Location + Width  bit1=0  base1=MSB of Input  bit0=17  base0=LSB of Input  dbl_ovrd=off  block_type=slice
  force1 : xbsIndex_r4/Reinterpret  force_arith_type=on  arith_type="Signed  (2's comp)"  force_bin_pt=on  bin_pt=35  block_type=reinterpret
  force2 : xbsIndex_r4/Reinterpret  force_arith_type=off  arith_type="Signed  (2's comp)"  force_bin_pt=on  bin_pt=35  block_type=reinterpret
  tweak_op : xbsIndex_r4/Logical  logical_function=AND  inputs=2  en=off  latency=0  precision=Full  arith_type=Unsigned  n_bits=8  bin_pt=2  align_bp=on  dbl_ovrd=off  block_type=logical
  out : Outport
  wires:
  tweak_op/1 -> Concat/2
  Constant/1 -> tweak_op/2
  bit/1 -> tweak_op/1
  almost_half/1 -> force2/1
  in/1 -> Reinterpret/1, bit/1
  Concat/1 -> force1/1
  Reinterpret/1 -> Concat/1
  force1/1 -> adder/1
  force2/1 -> adder/2
  adder/1 -> out/1

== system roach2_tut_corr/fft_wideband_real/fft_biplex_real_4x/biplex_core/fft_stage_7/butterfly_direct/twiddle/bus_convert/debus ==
  bus_in : Inport
  reinterpret{1..8} (8 alike) : xbsIndex_r4/Reinterpret  force_arith_type=on  arith_type="Signed  (2's comp)"  force_bin_pt=on  bin_pt=34  block_type=reinterpret
  slice1 : xbsIndex_r4/Slice  nbits=37  boolean_output=off  mode=Upper Bit Location + Width  bit1=-259  base1=MSB of Input  bit0=0  base0=LSB of Input  dbl_ovrd=off  block_type=slice
  slice2 : xbsIndex_r4/Slice  nbits=37  boolean_output=off  mode=Upper Bit Location + Width  bit1=-222  base1=MSB of Input  bit0=0  base0=LSB of Input  dbl_ovrd=off  block_type=slice
  slice3 : xbsIndex_r4/Slice  nbits=37  boolean_output=off  mode=Upper Bit Location + Width  bit1=-185  base1=MSB of Input  bit0=0  base0=LSB of Input  dbl_ovrd=off  block_type=slice
  slice4 : xbsIndex_r4/Slice  nbits=37  boolean_output=off  mode=Upper Bit Location + Width  bit1=-148  base1=MSB of Input  bit0=0  base0=LSB of Input  dbl_ovrd=off  block_type=slice
  slice5 : xbsIndex_r4/Slice  nbits=37  boolean_output=off  mode=Upper Bit Location + Width  bit1=-111  base1=MSB of Input  bit0=0  base0=LSB of Input  dbl_ovrd=off  block_type=slice
  slice6 : xbsIndex_r4/Slice  nbits=37  boolean_output=off  mode=Upper Bit Location + Width  bit1=-74  base1=MSB of Input  bit0=0  base0=LSB of Input  dbl_ovrd=off  block_type=slice
  slice7 : xbsIndex_r4/Slice  nbits=37  boolean_output=off  mode=Upper Bit Location + Width  bit1=-37  base1=MSB of Input  bit0=0  base0=LSB of Input  dbl_ovrd=off  block_type=slice
  slice8 : xbsIndex_r4/Slice  nbits=37  boolean_output=off  mode=Upper Bit Location + Width  bit1=0  base1=MSB of Input  bit0=0  base0=LSB of Input  dbl_ovrd=off  block_type=slice
  msb_out8 : Outport
  out7 : Outport  Port=2
  out6 : Outport  Port=3
  out5 : Outport  Port=4
  out4 : Outport  Port=5
  out3 : Outport  Port=6
  out2 : Outport  Port=7
  lsb_out1 : Outport  Port=8
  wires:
  bus_in/1 -> slice8/1, slice7/1, slice6/1, slice5/1, slice4/1, slice3/1, slice2/1, slice1/1
  slice8/1 -> reinterpret8/1
  reinterpret8/1 -> msb_out8/1
  slice7/1 -> reinterpret7/1
  reinterpret7/1 -> out7/1
  slice6/1 -> reinterpret6/1
  reinterpret6/1 -> out6/1
  slice5/1 -> reinterpret5/1
  reinterpret5/1 -> out5/1
  slice4/1 -> reinterpret4/1
  reinterpret4/1 -> out4/1
  slice3/1 -> reinterpret3/1
  reinterpret3/1 -> out3/1
  slice2/1 -> reinterpret2/1
  reinterpret2/1 -> out2/1
  slice1/1 -> reinterpret1/1
  reinterpret1/1 -> lsb_out1/1
